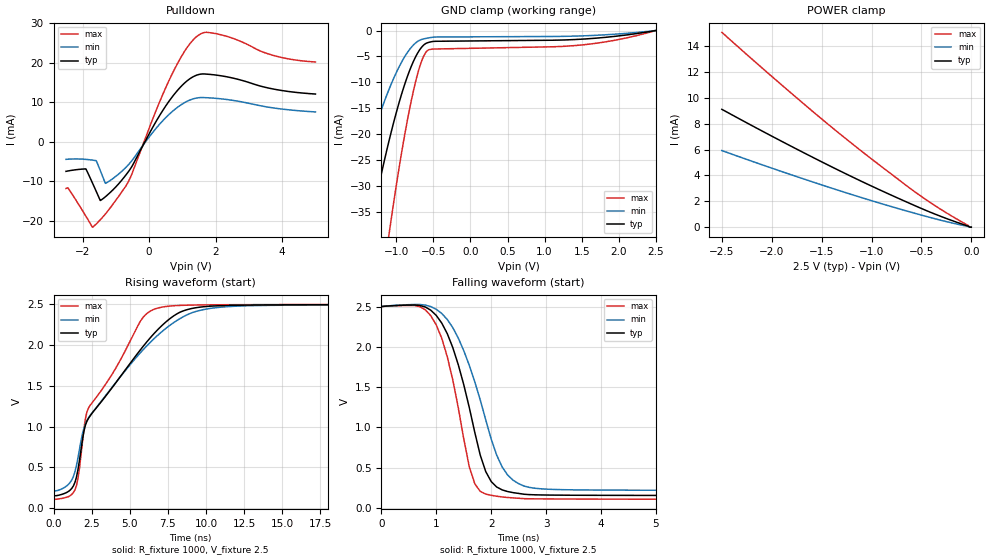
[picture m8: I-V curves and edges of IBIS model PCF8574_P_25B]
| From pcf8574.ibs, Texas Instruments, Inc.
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[Model]   PCF8574_P_25B
Model_type  I/O_open_drain
Vinl=.75
Vinh=1.75
Enable   Active-Low
Vref =   2.5
Rref =   4700
Cref =   10p
Vmeas =   1.25
| variable   typ   min   max
C_comp   1.36pF   1.26pF   1.48pF
| C_pulldown   1.29pF   1.18pF   1.50pF
| C_tri-state   1.36pF   1.26pF   1.48pF
[Temperature Range]   40   100   -40
| Ambient temperature   25   85   -40
[Voltage range]   2.5   2.5   2.5
[Pullup Reference]   2.5   2.5   2.5
[POWER Clamp Reference]   2.5   2.5   2.5
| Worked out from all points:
|   slope of the pulldown table from 0 to 0.375 V, typ, clamps not added: 68.6 ohm
|   POWER clamp passes 1 mA (typ) near -0.36 V on its own axis
|   rising waveform, R_fixture 1000, V_fixture 2.5: 20-80 % time 4.34ns typ, 4.73ns min, 3.19ns max; typ from 0.152 V to 2.5 V
|   falling waveform, R_fixture 1000, V_fixture 2.5: 20-80 % time 540ps typ, 650ps min, 443ps max; typ from 2.5 V to 0.152 V
[GND Clamp]
| PCF8574_P_25B
|   Voltage   I(typ)   I(min)   I(max)
-2.5V     -161mA     -117.5mA   -239.6mA
-1.57V    -57.05mA   -39.19mA   -93.82mA
-1.535V   -53.42mA   -36.48mA   -89.4mA
-1.36V    -38.53mA   -23.37mA   -68.09mA
-1.295V   -33.95mA   -19.26mA   -60.57mA
-1.09V    -20.83mA   -11.08mA   -38.56mA
-870mV    -9.688mA   -4.679mA   -18.84mA
-695mV    -3.955mA   -1.953mA   -7.493mA
-610mV    -2.572mA   -1.553mA   -4.406mA
-530mV    -2.173mA   -1.337mA   -3.613mA
1.415V    -1.736mA   -1.077mA   -2.9mA
2.5V      277.1pA    450.8pA    79.62pA
[POWER Clamp]
| PCF8574_P_25B
|   Voltage   I(typ)   I(min)   I(max)
-2.5V     9.108mA    5.921mA    15.06mA
-1.66V    5.677mA    3.674mA    9.405mA
-1.07V    3.43mA     2.213mA    5.693mA
-480mV    1.378mA    889.3uA    2.266mA
-255mV    685.6uA    439.5uA    1.134mA
-30mV     75.66uA    48.11uA    125.7uA
-15mV     0A         0A         0A
-31.15fV  0A         0A         0A
[Pulldown]
| PCF8574_P_25B
|   Voltage   I(typ)   I(min)   I(max)
-2.5V     -7.476mA   -4.438mA   -11.82mA
-1.905V   -6.851mA   -4.444mA   -18.79mA
-1.705V   -10.41mA   -4.627mA   -21.61mA
-1.59V    -12.57mA   -4.784mA   -20.8mA
-1.47V    -14.85mA   -7.249mA   -19.76mA
-1.38V    -14.35mA   -9.164mA   -18.92mA
-1.28V    -13.66mA   -10.38mA   -17.91mA
-590mV    -7.162mA   -5.481mA   -9.498mA
290mV     6.322mA    4.232mA    9.624mA
840mV     12.91mA    8.664mA    19.64mA
1.555V    17.16mA    11.22mA    27.38mA
5V        12.11mA    7.575mA    20.22mA
[Ramp]
| PCF8574_P_25B
| variable   typ   min   max
dV/dt_r   1.41/4.34E-09   1.37/4.73E-09   1.44/3.19E-09
dV/dt_f   1.42/5.45E-10   1.39/6.60E-10   1.44/4.44E-10
R_load = 1000
[Rising Waveform]
| PCF8574_P_25B
R_fixture =   1000
C_fixture =   0
L_fixture =   0
V_fixture =   2.5
V_fixture_min = 2.5
V_fixture_max = 2.5
|   Time   V(typ)   V(min)   V(max)
0s        152.4mV    214.5mV    107.8mV
900ps     194.3mV    276.7mV    133.8mV
1.4ns     311.6mV    441.4mV    221.5mV
1.6ns     467.4mV    612.8mV    358.4mV
2.2ns     1.07V      1.077V     1.185V
5.7ns     1.943V     1.907V     2.296V
8.2ns     2.396V     2.316V     2.488V
10.9ns    2.485V     2.466V     2.497V
18.3ns    2.498V     2.495V     2.499V
269.9ns   2.5V       2.5V       2.5V
[Falling Waveform]
| PCF8574_P_25B
R_fixture =   1000
C_fixture =   0
L_fixture =   0
V_fixture =   2.5
V_fixture_min = 2.5
V_fixture_max = 2.5
|   Time   V(typ)   V(min)   V(max)
0s        2.5V       2.5V       2.5V
800ps     2.494V     2.518V     2.459V
1ns       2.389V     2.465V     2.27V
1.2ns     2.163V     2.339V     1.876V
1.6ns     1.249V     1.772V     512.7mV
1.7ns     940.8mV    1.568V     302.5mV
1.9ns     452.7mV    1.095V     173.1mV
2.2ns     224.7mV    509.1mV    137.3mV
2.7ns     166.2mV    255.2mV    114.5mV
269.9ns   152.4mV    214.5mV    107.8mV
